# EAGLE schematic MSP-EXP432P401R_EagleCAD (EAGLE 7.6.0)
AUTHOR: Mike Stein; REV: 2.1

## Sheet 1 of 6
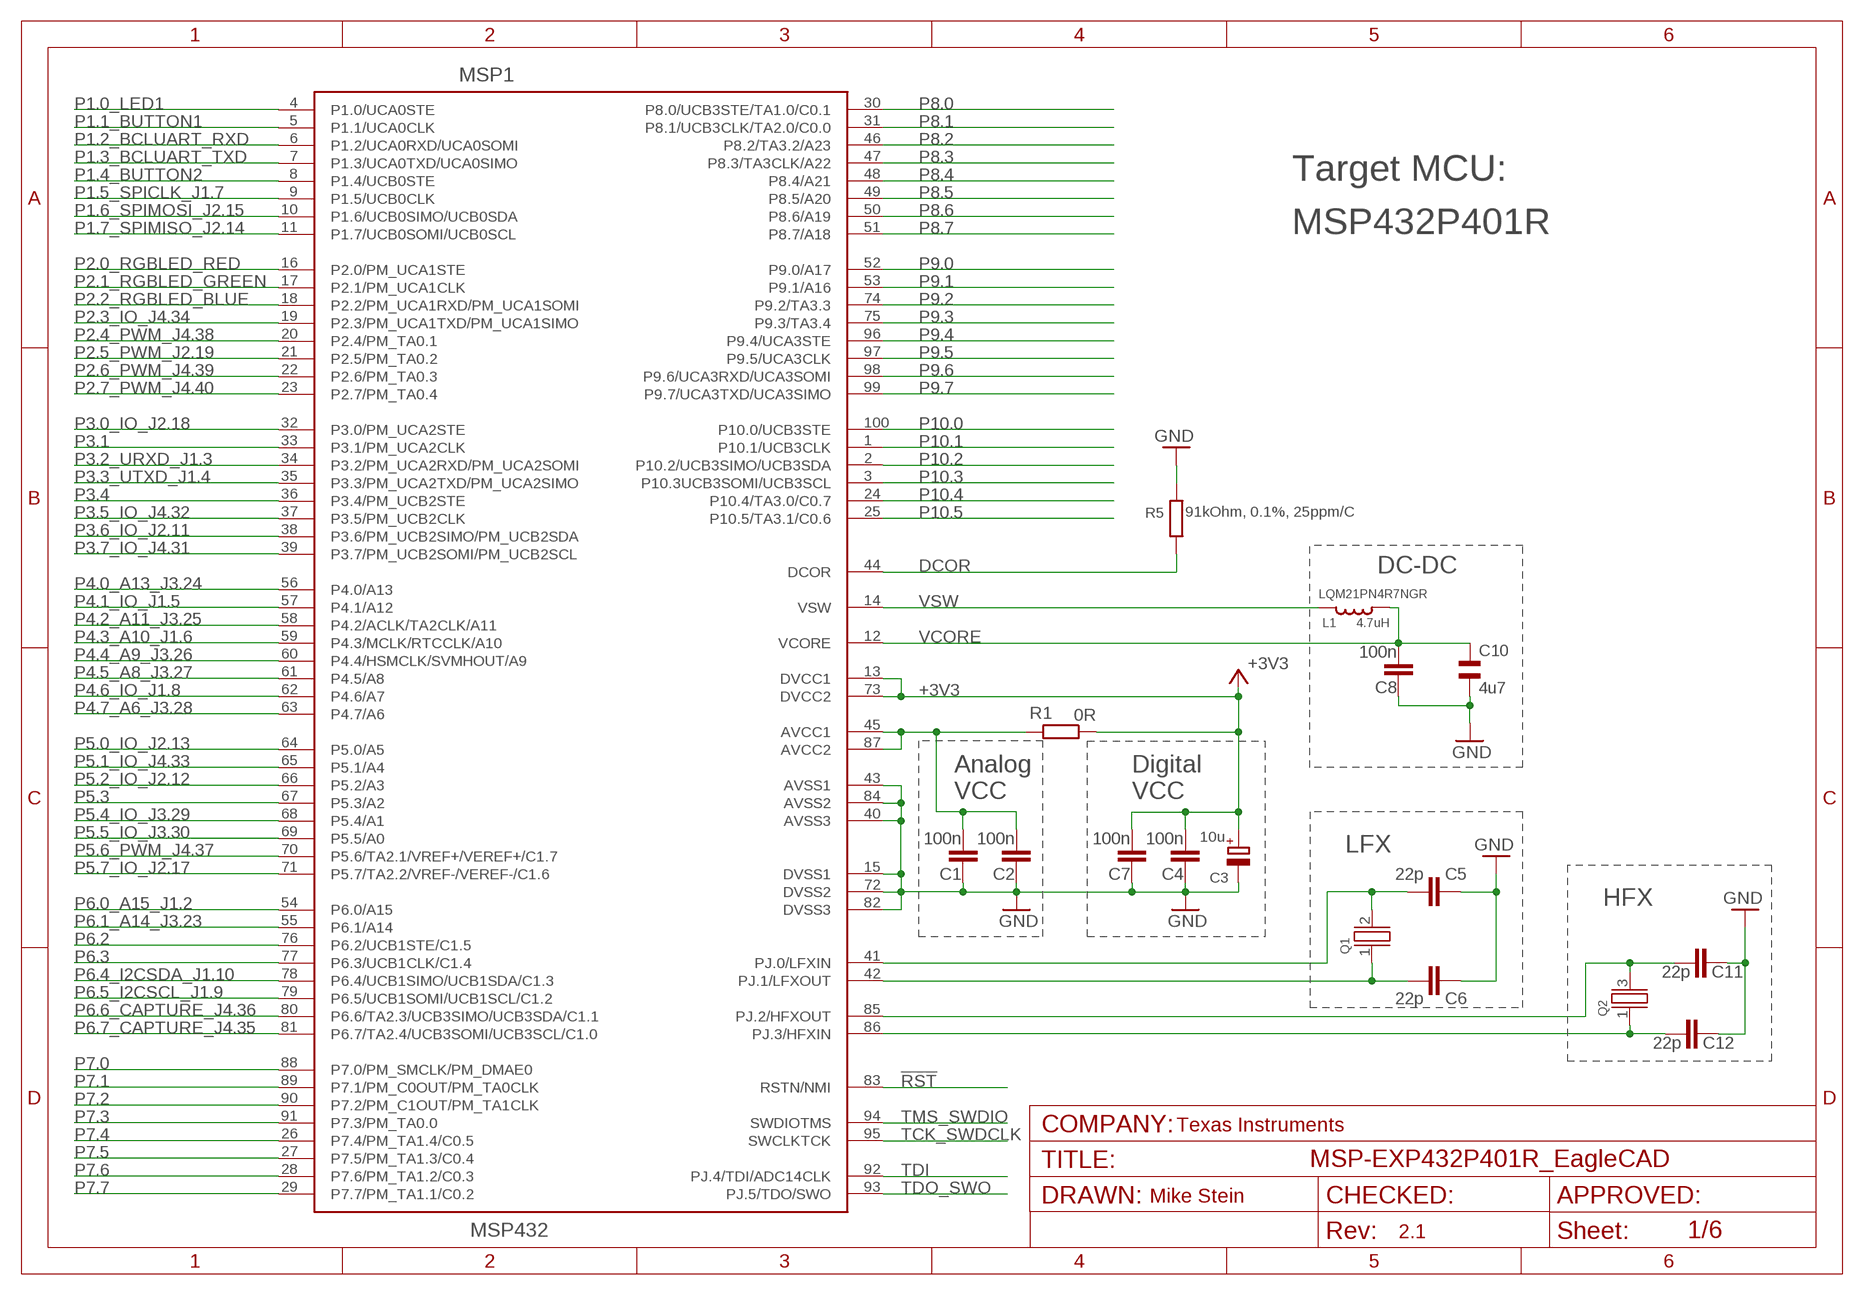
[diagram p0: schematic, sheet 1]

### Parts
C1  100n  C-EUCM0402  [0402]
C2  100n  C-EUCM0402  [0402]
C3  10u  CPOL-EUA/3216-18R  [A/3216-18R]
C4  100n  C-EUCM0402  [0402]
C5  22p  C-EUCM0402  [0402]
C6  22p  C-EUCM0402  [0402]
C7  100n  C-EUCM0402  [0402]
C8  100n  C-EUCM0402  [0402]
C10  4u7  CSMD0805  [CSMD0805]
C11  22p  C-EUCM0402  [0402]
C12  22p  C-EUCM0402  [0402]
L1  4.7uH  LQM2MP_G0  [0806]
MSP1  MSP432  [PZ100]
Q1  CRYSTALLF_GENERAL  [LF_XTAL]
Q2  CRYSTALEPSON_FA-238  [FA-238]
R1  0R  R-EU_RM0402  [0402]
R5  91kOhm, 0.1%, 25ppm/C  R_0805  [0805]

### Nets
!RST: MSP1.83(RSTN/NMI) ; also sheet 2,3
+3V3: C3.+ C4.1 C7.1 MSP1.13(DVCC1) MSP1.73(DVCC2) R1.1 ; also sheet 2,3
DCOR: MSP1.44(DCOR) R5.1
N$6: C1.1 C2.1 MSP1.45(AVCC1) MSP1.87(AVCC2) R1.2
N$34: C6.1 MSP1.42(PJ.1/LFXOUT) Q1.1
N$38: C5.1 MSP1.41(PJ.0/LFXIN) Q1.2
P1.0_LED1: MSP1.4(P1.0/UCA0STE) ; also sheet 2
P1.1_BUTTON1: MSP1.5(P1.1/UCA0CLK) ; also sheet 2
P1.2_BCLUART_RXD: MSP1.6(P1.2/UCA0RXD/UCA0SOMI) ; also sheet 3
P1.3_BCLUART_TXD: MSP1.7(P1.3/UCA0TXD/UCA0SIMO) ; also sheet 3
P1.4_BUTTON2: MSP1.8(P1.4/UCB0STE) ; also sheet 2
P1.5_SPICLK_J1.7: MSP1.9(P1.5/UCB0CLK) ; also sheet 3
P1.6_SPIMOSI_J2.15: MSP1.10(P1.6/UCB0SIMO/UCB0SDA) ; also sheet 3
P1.7_SPIMISO_J2.14: MSP1.11(P1.7/UCB0SOMI/UCB0SCL) ; also sheet 3
P2.0_RGBLED_RED: MSP1.16(P2.0/PM_UCA1STE) ; also sheet 2
P2.1_RGBLED_GREEN: MSP1.17(P2.1/PM_UCA1CLK) ; also sheet 2
P2.2_RGBLED_BLUE: MSP1.18(P2.2/PM_UCA1RXD/PM_UCA1SOMI) ; also sheet 2
P2.3_IO_J4.34: MSP1.19(P2.3/PM_UCA1TXD/PM_UCA1SIMO) ; also sheet 3
P2.4_PWM_J4.38: MSP1.20(P2.4/PM_TA0.1) ; also sheet 3
P2.5_PWM_J2.19: MSP1.21(P2.5/PM_TA0.2) ; also sheet 3
P2.6_PWM_J4.39: MSP1.22(P2.6/PM_TA0.3) ; also sheet 3
P2.7_PWM_J4.40: MSP1.23(P2.7/PM_TA0.4) ; also sheet 3
P3.0_IO_J2.18: MSP1.32(P3.0/PM_UCA2STE) ; also sheet 3
P3.1: MSP1.33(P3.1/PM_UCA2CLK)
P3.2_URXD_J1.3: MSP1.34(P3.2/PM_UCA2RXD/PM_UCA2SOMI) ; also sheet 3
P3.3_UTXD_J1.4: MSP1.35(P3.3/PM_UCA2TXD/PM_UCA2SIMO) ; also sheet 3
P3.4: MSP1.36(P3.4/PM_UCB2STE)
P3.5_IO_J4.32: MSP1.37(P3.5/PM_UCB2CLK) ; also sheet 3
P3.6_IO_J2.11: MSP1.38(P3.6/PM_UCB2SIMO/PM_UCB2SDA) ; also sheet 3
P3.7_IO_J4.31: MSP1.39(P3.7/PM_UCB2SOMI/PM_UCB2SCL) ; also sheet 3
P4.0_A13_J3.24: MSP1.56(P4.0/A13) ; also sheet 3
P4.1_IO_J1.5: MSP1.57(P4.1/A12) ; also sheet 3
P4.2_A11_J3.25: MSP1.58(P4.2/ACLK/TA2CLK/A11) ; also sheet 3
P4.3_A10_J1.6: MSP1.59(P4.3/MCLK/RTCCLK/A10) ; also sheet 3
P4.4_A9_J3.26: MSP1.60(P4.4/HSMCLK/SVMHOUT/A9) ; also sheet 3
P4.5_A8_J3.27: MSP1.61(P4.5/A8) ; also sheet 3
P4.6_IO_J1.8: MSP1.62(P4.6/A7) ; also sheet 3
P4.7_A6_J3.28: MSP1.63(P4.7/A6) ; also sheet 3
P5.0_IO_J2.13: MSP1.64(P5.0/A5) ; also sheet 3
P5.1_IO_J4.33: MSP1.65(P5.1/A4) ; also sheet 3
P5.2/XT2IN: C12.1 MSP1.86(PJ.3/HFXIN) Q2.1
P5.2_IO_J2.12: MSP1.66(P5.2/A3) ; also sheet 3
P5.3: MSP1.67(P5.3/A2) ; also sheet 3
P5.3/XT2OUT: C11.1 MSP1.85(PJ.2/HFXOUT) Q2.3
P5.4_IO_J3.29: MSP1.68(P5.4/A1) ; also sheet 3
P5.5_IO_J3.30: MSP1.69(P5.5/A0) ; also sheet 3
P5.6_PWM_J4.37: MSP1.70(P5.6/TA2.1/VREF+/VEREF+/C1.7) ; also sheet 3
P5.7_IO_J2.17: MSP1.71(P5.7/TA2.2/VREF-/VEREF-/C1.6) ; also sheet 3
P6.0_A15_J1.2: MSP1.54(P6.0/A15) ; also sheet 3
P6.1_A14_J3.23: MSP1.55(P6.1/A14) ; also sheet 3
P6.2: MSP1.76(P6.2/UCB1STE/C1.5) ; also sheet 3
P6.3: MSP1.77(P6.3/UCB1CLK/C1.4) ; also sheet 3
P6.4_I2CSDA_J1.10: MSP1.78(P6.4/UCB1SIMO/UCB1SDA/C1.3) ; also sheet 3
P6.5_I2CSCL_J1.9: MSP1.79(P6.5/UCB1SOMI/UCB1SCL/C1.2) ; also sheet 3
P6.6_CAPTURE_J4.36: MSP1.80(P6.6/TA2.3/UCB3SIMO/UCB3SDA/C1.1) ; also sheet 3
P6.7_CAPTURE_J4.35: MSP1.81(P6.7/TA2.4/UCB3SOMI/UCB3SCL/C1.0) ; also sheet 3
P7.0: MSP1.88(P7.0/PM_SMCLK/PM_DMAE0) ; also sheet 3
P7.1: MSP1.89(P7.1/PM_C0OUT/PM_TA0CLK) ; also sheet 3
P7.2: MSP1.90(P7.2/PM_C1OUT/PM_TA1CLK) ; also sheet 3
P7.3: MSP1.91(P7.3/PM_TA0.0) ; also sheet 3
P7.4: MSP1.26(P7.4/PM_TA1.4/C0.5) ; also sheet 3
P7.5: MSP1.27(P7.5/PM_TA1.3/C0.4) ; also sheet 3
P7.6: MSP1.28(P7.6/PM_TA1.2/C0.3) ; also sheet 3
P7.7: MSP1.29(P7.7/PM_TA1.1/C0.2) ; also sheet 3
P8.0: MSP1.30(P8.0/UCB3STE/TA1.0/C0.1) ; also sheet 3
P8.1: MSP1.31(P8.1/UCB3CLK/TA2.0/C0.0)
P8.2: MSP1.46(P8.2/TA3.2/A23) ; also sheet 3
P8.3: MSP1.47(P8.3/TA3CLK/A22) ; also sheet 3
P8.4: MSP1.48(P8.4/A21) ; also sheet 3
P8.5: MSP1.49(P8.5/A20) ; also sheet 3
P8.6: MSP1.50(P8.6/A19) ; also sheet 3
P8.7: MSP1.51(P8.7/A18) ; also sheet 3
P9.0: MSP1.52(P9.0/A17) ; also sheet 3
P9.1: MSP1.53(P9.1/A16) ; also sheet 3
P9.2: MSP1.74(P9.2/TA3.3) ; also sheet 3
P9.3: MSP1.75(P9.3/TA3.4) ; also sheet 3
P9.4: MSP1.96(P9.4/UCA3STE) ; also sheet 3
P9.5: MSP1.97(P9.5/UCA3CLK) ; also sheet 3
P9.6: MSP1.98(P9.6/UCA3RXD/UCA3SOMI) ; also sheet 3
P9.7: MSP1.99(P9.7/UCA3TXD/UCA3SIMO) ; also sheet 3
P10.0: MSP1.100(P10.0/UCB3STE) ; also sheet 3
P10.1: MSP1.1(P10.1/UCB3CLK) ; also sheet 3
P10.2: MSP1.2(P10.2/UCB3SIMO/UCB3SDA) ; also sheet 3
P10.3: MSP1.3(P10.3UCB3SOMI/UCB3SCL) ; also sheet 3
P10.4: MSP1.24(P10.4/TA3.0/C0.7) ; also sheet 3
P10.5: MSP1.25(P10.5/TA3.1/C0.6) ; also sheet 3
TCK_SWDCLK: MSP1.95(SWCLKTCK) ; also sheet 3
TDI: MSP1.92(PJ.4/TDI/ADC14CLK) ; also sheet 3
TDO_SWO: MSP1.93(PJ.5/TDO/SWO) ; also sheet 3
TMS_SWDIO: MSP1.94(SWDIOTMS) ; also sheet 3
VCORE: C8.1 C10.1 L1.1 MSP1.12(VCORE)
VSW: L1.2 MSP1.14(VSW)
XDS-GND: C1.2 C2.2 C3.- C4.2 C5.2 C6.2 C7.2 C8.2 C10.2 C11.2 C12.2 MSP1.15(DVSS1) MSP1.40(AVSS3) MSP1.43(AVSS1) MSP1.72(DVSS2) MSP1.82(DVSS3) MSP1.84(AVSS2) R5.2 ; supply symbol labelled GND ; also sheet 2,3

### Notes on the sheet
- Target MCU:
- MSP432P401R
- DC-DC
- LQM21PN4R7NGR
- Analog | Digital
- VCC | VCC
- LFX
- HFX
- Texas Instruments

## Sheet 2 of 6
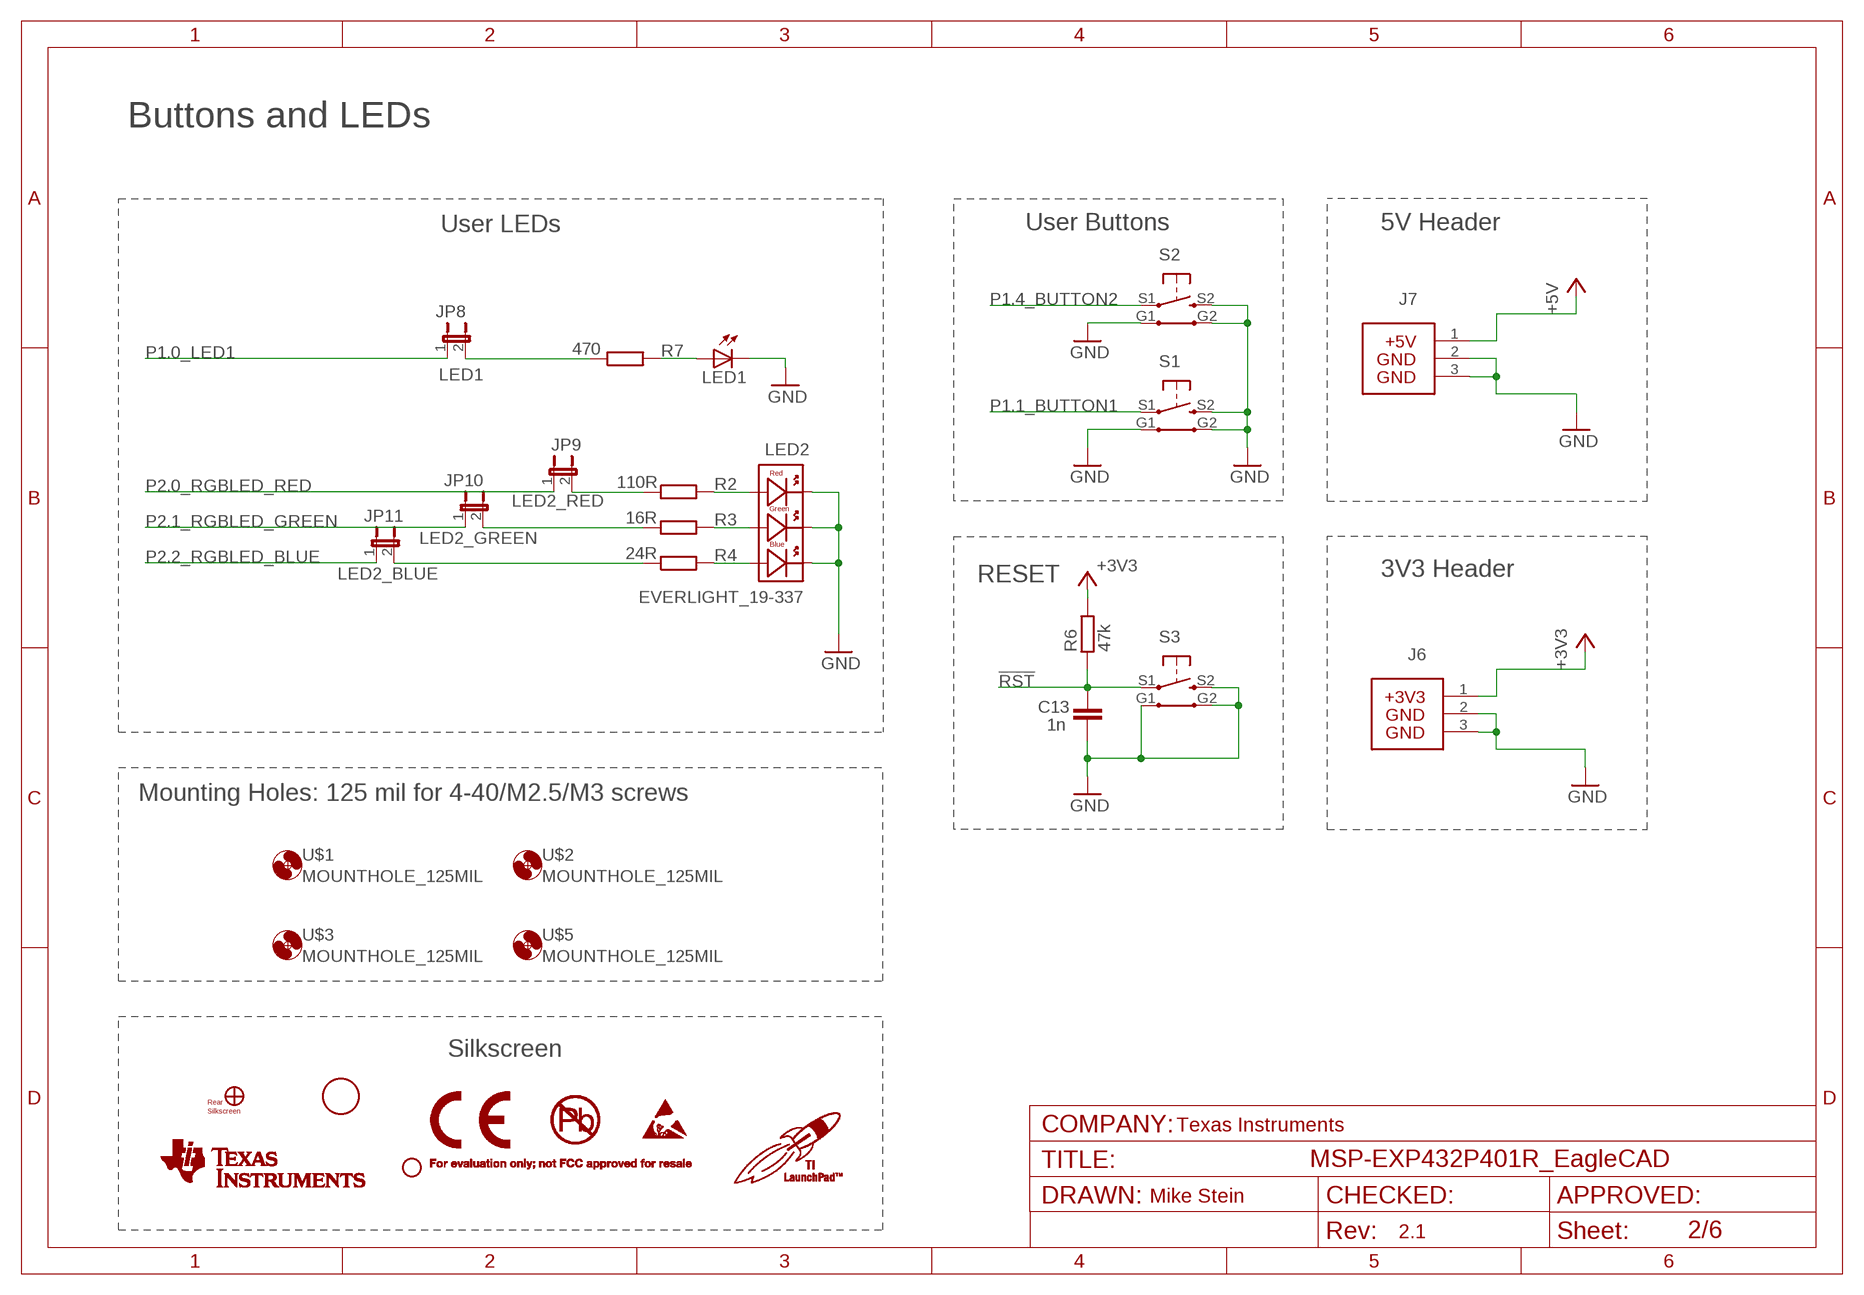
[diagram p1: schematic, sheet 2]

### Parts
C13  1n  C-EUCM0402  [0402]
J6  HEADER 1X03  BP_HEADERS_PWR_3V3100-TH  [3PIN_PWR_3V3]
J7  BP_HEADERS_PWR_5V  [3PIN_PWR_5V]
JP8  LED1  JP1M  [JP1M]
JP9  LED2_RED  JP1M  [JP1M]
JP10  LED2_GREEN  JP1M  [JP1M]
JP11  LED2_BLUE  JP1M  [JP1M]
LED1  LEDCHIPLED_0603  [CHIPLED_0603]
LED2  EVERLIGHT_19-337  [RGB_LED]
R2  110R  R-EU_RM0402  [0402]
R3  16R  R-EU_RM0402  [0402]
R4  24R  R-EU_RM0402  [0402]
R6  47k  R-EU_RM0402  [0402]
R7  470  R-EU_RM0402  [0402]
S1  TS-1188E  [TS-1188E]
S2  TS-1188E  [TS-1188E]
S3  TS-1188E  [TS-1188E]
U$1  MOUNTHOLE_125MIL  [MOUNTHOLE_125MIL]
U$2  MOUNTHOLE_125MIL  [MOUNTHOLE_125MIL]
U$3  MOUNTHOLE_125MIL  [MOUNTHOLE_125MIL]
U$5  MOUNTHOLE_125MIL  [MOUNTHOLE_125MIL]
U$7  MIKE_TM  [MIKE_TM]
U$8  P401R_REARSILK_REV2_1  [P401R_REARSILK_REV2_1]
U$9  REAR_TILOGO  [REAR_TILOGO]
U$10  COMPLIANCE_SUITESYMBOLONLY  [EVM_COMPLIANCESUITE_SYMBOLONLY]
U$11  COMPLIANCE_FCC_TEXTREAR  [COMPLIANCE_FCC_TEXT]
U$12  LOGO-ROCKET  [LOGO-ROCKET]
U$13  P401R_SILKLABEL  [SILKLABELUPDATED]

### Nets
!RST: C13.1 R6.1 S3.S1(P) ; also sheet 1,3
+3V3: J6.1 R6.2 ; also sheet 1,3
+5V [Power]: J7.1 ; also sheet 3
N$8: JP9.2 R2.1
N$9: LED2.5(RA) R2.2
N$10: LED2.6(GA) R3.2
N$11: LED2.4(BA) R4.2
N$17: LED1.A R7.2
N$19: JP10.2 R3.1
N$25: JP11.2 R4.1
N$29: JP8.2 R7.1
P1.0_LED1: JP8.1 ; also sheet 1
P1.1_BUTTON1: S1.S1(P) ; also sheet 1
P1.4_BUTTON2: S2.S1(P) ; also sheet 1
P2.0_RGBLED_RED: JP9.1 ; also sheet 1
P2.1_RGBLED_GREEN: JP10.1 ; also sheet 1
P2.2_RGBLED_BLUE: JP11.1 ; also sheet 1
XDS-GND: C13.2 J6.2 J6.3 J7.2 J7.3 LED1.C LED2.1(BC) LED2.2(RC) LED2.3(GC) S1.G1 S1.G2 S1.S2(S) S2.G1 S2.G2 S2.S2(S) S3.G1 S3.G2 S3.S2(S) ; supply symbol labelled GND ; also sheet 1,3

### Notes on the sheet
- Buttons and LEDs
- User LEDs | User Buttons | 5V Header
- RESET | 3V3 Header
- Mounting Holes: 125 mil for 4-40/M2.5/M3 screws
- Silkscreen
- Texas Instruments

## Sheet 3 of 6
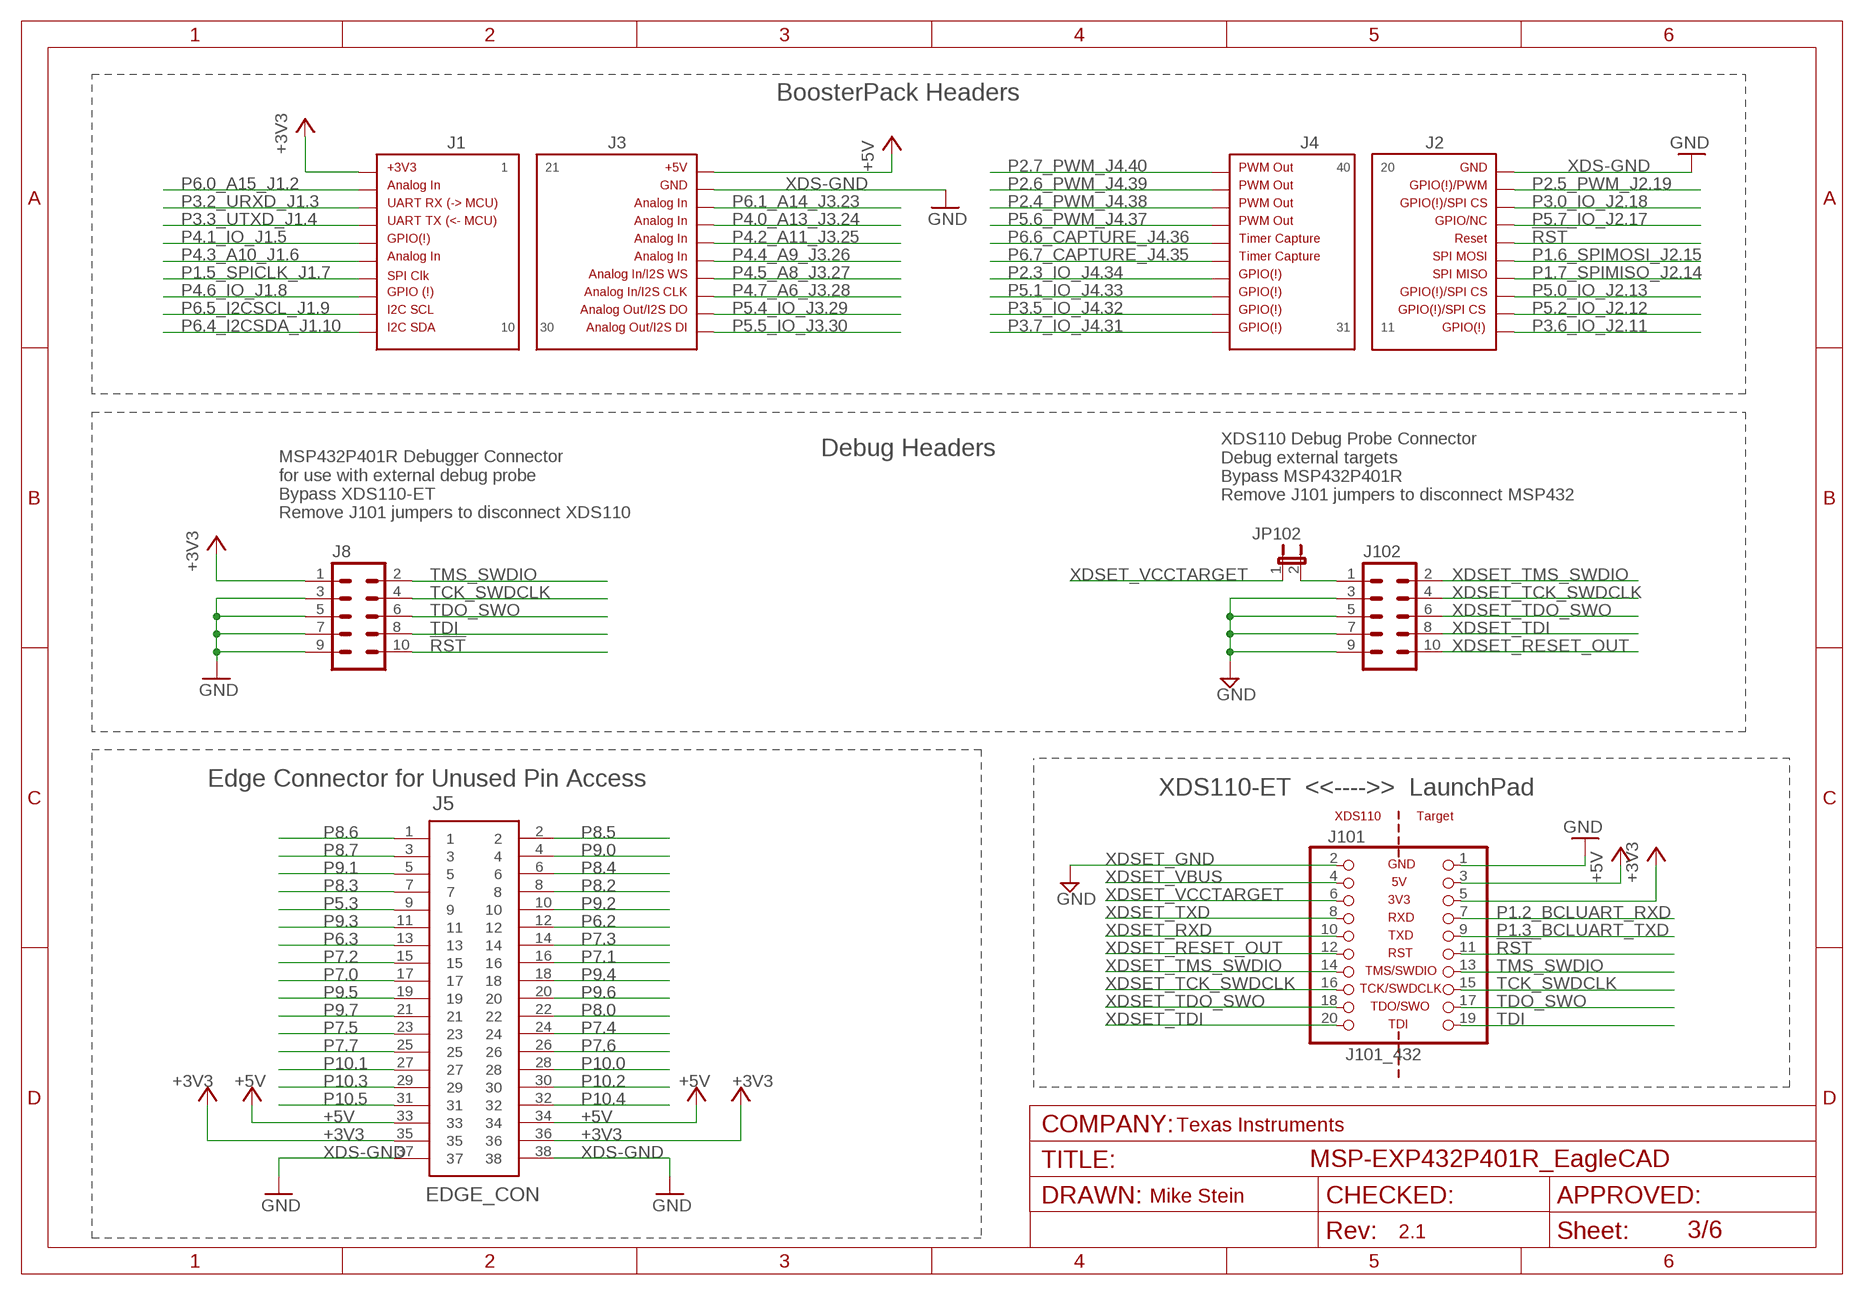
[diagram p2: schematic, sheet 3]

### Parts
J1  HEADER1X10-J1SILK_LABELS  [J1]
J2  HEADER1X10-J2SILK_LABELS  [J2]
J3  HEADER1X10-J3  [J3]
J4  HEADER1X10-J4SILK_LABELS  [J4]
J5  EDGE_CON  [BOTTOM_CONNECTOR]
J8  DEBUG_ARM-10  [ARM-10]
J101  J101_432  [J101_432]
J102  DEBUG_ARM-10  [ARM-10]
JP102  JP1M  [JP1M]

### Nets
!RST: J2.16 J8.10 J101.11 ; also sheet 1,2
+3V3: J1.1 J5.35 J5.36 J8.1 J101.5 ; also sheet 1,2
+5V [Power]: J3.21 J5.33 J5.34 J101.3 ; also sheet 2
N$1: J102.1 JP102.2
P1.2_BCLUART_RXD: J101.7 ; also sheet 1
P1.3_BCLUART_TXD: J101.9 ; also sheet 1
P1.5_SPICLK_J1.7: J1.7 ; also sheet 1
P1.6_SPIMOSI_J2.15: J2.15 ; also sheet 1
P1.7_SPIMISO_J2.14: J2.14 ; also sheet 1
P2.3_IO_J4.34: J4.34 ; also sheet 1
P2.4_PWM_J4.38: J4.38 ; also sheet 1
P2.5_PWM_J2.19: J2.19 ; also sheet 1
P2.6_PWM_J4.39: J4.39 ; also sheet 1
P2.7_PWM_J4.40: J4.40 ; also sheet 1
P3.0_IO_J2.18: J2.18 ; also sheet 1
P3.2_URXD_J1.3: J1.3 ; also sheet 1
P3.3_UTXD_J1.4: J1.4 ; also sheet 1
P3.5_IO_J4.32: J4.32 ; also sheet 1
P3.6_IO_J2.11: J2.11 ; also sheet 1
P3.7_IO_J4.31: J4.31 ; also sheet 1
P4.0_A13_J3.24: J3.24 ; also sheet 1
P4.1_IO_J1.5: J1.5 ; also sheet 1
P4.2_A11_J3.25: J3.25 ; also sheet 1
P4.3_A10_J1.6: J1.6 ; also sheet 1
P4.4_A9_J3.26: J3.26 ; also sheet 1
P4.5_A8_J3.27: J3.27 ; also sheet 1
P4.6_IO_J1.8: J1.8 ; also sheet 1
P4.7_A6_J3.28: J3.28 ; also sheet 1
P5.0_IO_J2.13: J2.13 ; also sheet 1
P5.1_IO_J4.33: J4.33 ; also sheet 1
P5.2_IO_J2.12: J2.12 ; also sheet 1
P5.3: J5.9 ; also sheet 1
P5.4_IO_J3.29: J3.29 ; also sheet 1
P5.5_IO_J3.30: J3.30 ; also sheet 1
P5.6_PWM_J4.37: J4.37 ; also sheet 1
P5.7_IO_J2.17: J2.17 ; also sheet 1
P6.0_A15_J1.2: J1.2 ; also sheet 1
P6.1_A14_J3.23: J3.23 ; also sheet 1
P6.2: J5.12 ; also sheet 1
P6.3: J5.13 ; also sheet 1
P6.4_I2CSDA_J1.10: J1.10 ; also sheet 1
P6.5_I2CSCL_J1.9: J1.9 ; also sheet 1
P6.6_CAPTURE_J4.36: J4.36 ; also sheet 1
P6.7_CAPTURE_J4.35: J4.35 ; also sheet 1
P7.0: J5.17 ; also sheet 1
P7.1: J5.16 ; also sheet 1
P7.2: J5.15 ; also sheet 1
P7.3: J5.14 ; also sheet 1
P7.4: J5.24 ; also sheet 1
P7.5: J5.23 ; also sheet 1
P7.6: J5.26 ; also sheet 1
P7.7: J5.25 ; also sheet 1
P8.0: J5.22 ; also sheet 1
P8.2: J5.8 ; also sheet 1
P8.3: J5.7 ; also sheet 1
P8.4: J5.6 ; also sheet 1
P8.5: J5.2 ; also sheet 1
P8.6: J5.1 ; also sheet 1
P8.7: J5.3 ; also sheet 1
P9.0: J5.4 ; also sheet 1
P9.1: J5.5 ; also sheet 1
P9.2: J5.10 ; also sheet 1
P9.3: J5.11 ; also sheet 1
P9.4: J5.18 ; also sheet 1
P9.5: J5.19 ; also sheet 1
P9.6: J5.20 ; also sheet 1
P9.7: J5.21 ; also sheet 1
P10.0: J5.28 ; also sheet 1
P10.1: J5.27 ; also sheet 1
P10.2: J5.30 ; also sheet 1
P10.3: J5.29 ; also sheet 1
P10.4: J5.32 ; also sheet 1
P10.5: J5.31 ; also sheet 1
TCK_SWDCLK: J8.4 J101.15 ; also sheet 1
TDI: J8.8 J101.19 ; also sheet 1
TDO_SWO: J8.6 J101.17 ; also sheet 1
TMS_SWDIO: J8.2 J101.13 ; also sheet 1
XDS-GND: J2.20 J3.22 J5.37 J5.38 J8.3 J8.5 J8.7 J8.9 J101.1 ; supply symbol labelled GND ; also sheet 1,2
XDSET_GND: J101.2 J102.3 J102.5 J102.7 J102.9 ; supply symbol labelled GND ; also sheet 4,5,6
XDSET_RESET_OUT: J101.12 J102.10 ; also sheet 4
XDSET_RXD: J101.10 ; also sheet 4
XDSET_TCK_SWDCLK: J101.16 J102.4 ; also sheet 4
XDSET_TDI: J101.20 J102.8 ; also sheet 4
XDSET_TDO_SWO: J101.18 J102.6 ; also sheet 4
XDSET_TMS_SWDIO: J101.14 J102.2 ; also sheet 4
XDSET_TXD: J101.8 ; also sheet 4
XDSET_VBUS: J101.4 ; also sheet 4,5,6
XDSET_VCCTARGET: J101.6 JP102.1 ; also sheet 5

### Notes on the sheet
- BoosterPack Headers
- Debug Headers
- XDS110 Debug Probe Connector
  Debug external targets
  Bypass MSP432P401R
  Remove J101 jumpers to disconnect MSP432
- MSP432P401R Debugger Connector
  for use with external debug probe
  Bypass XDS110-ET
  Remove J101 jumpers to disconnect XDS110
- Edge Connector for Unused Pin Access
- XDS110-ET  <<---->>  LaunchPad
- Texas Instruments

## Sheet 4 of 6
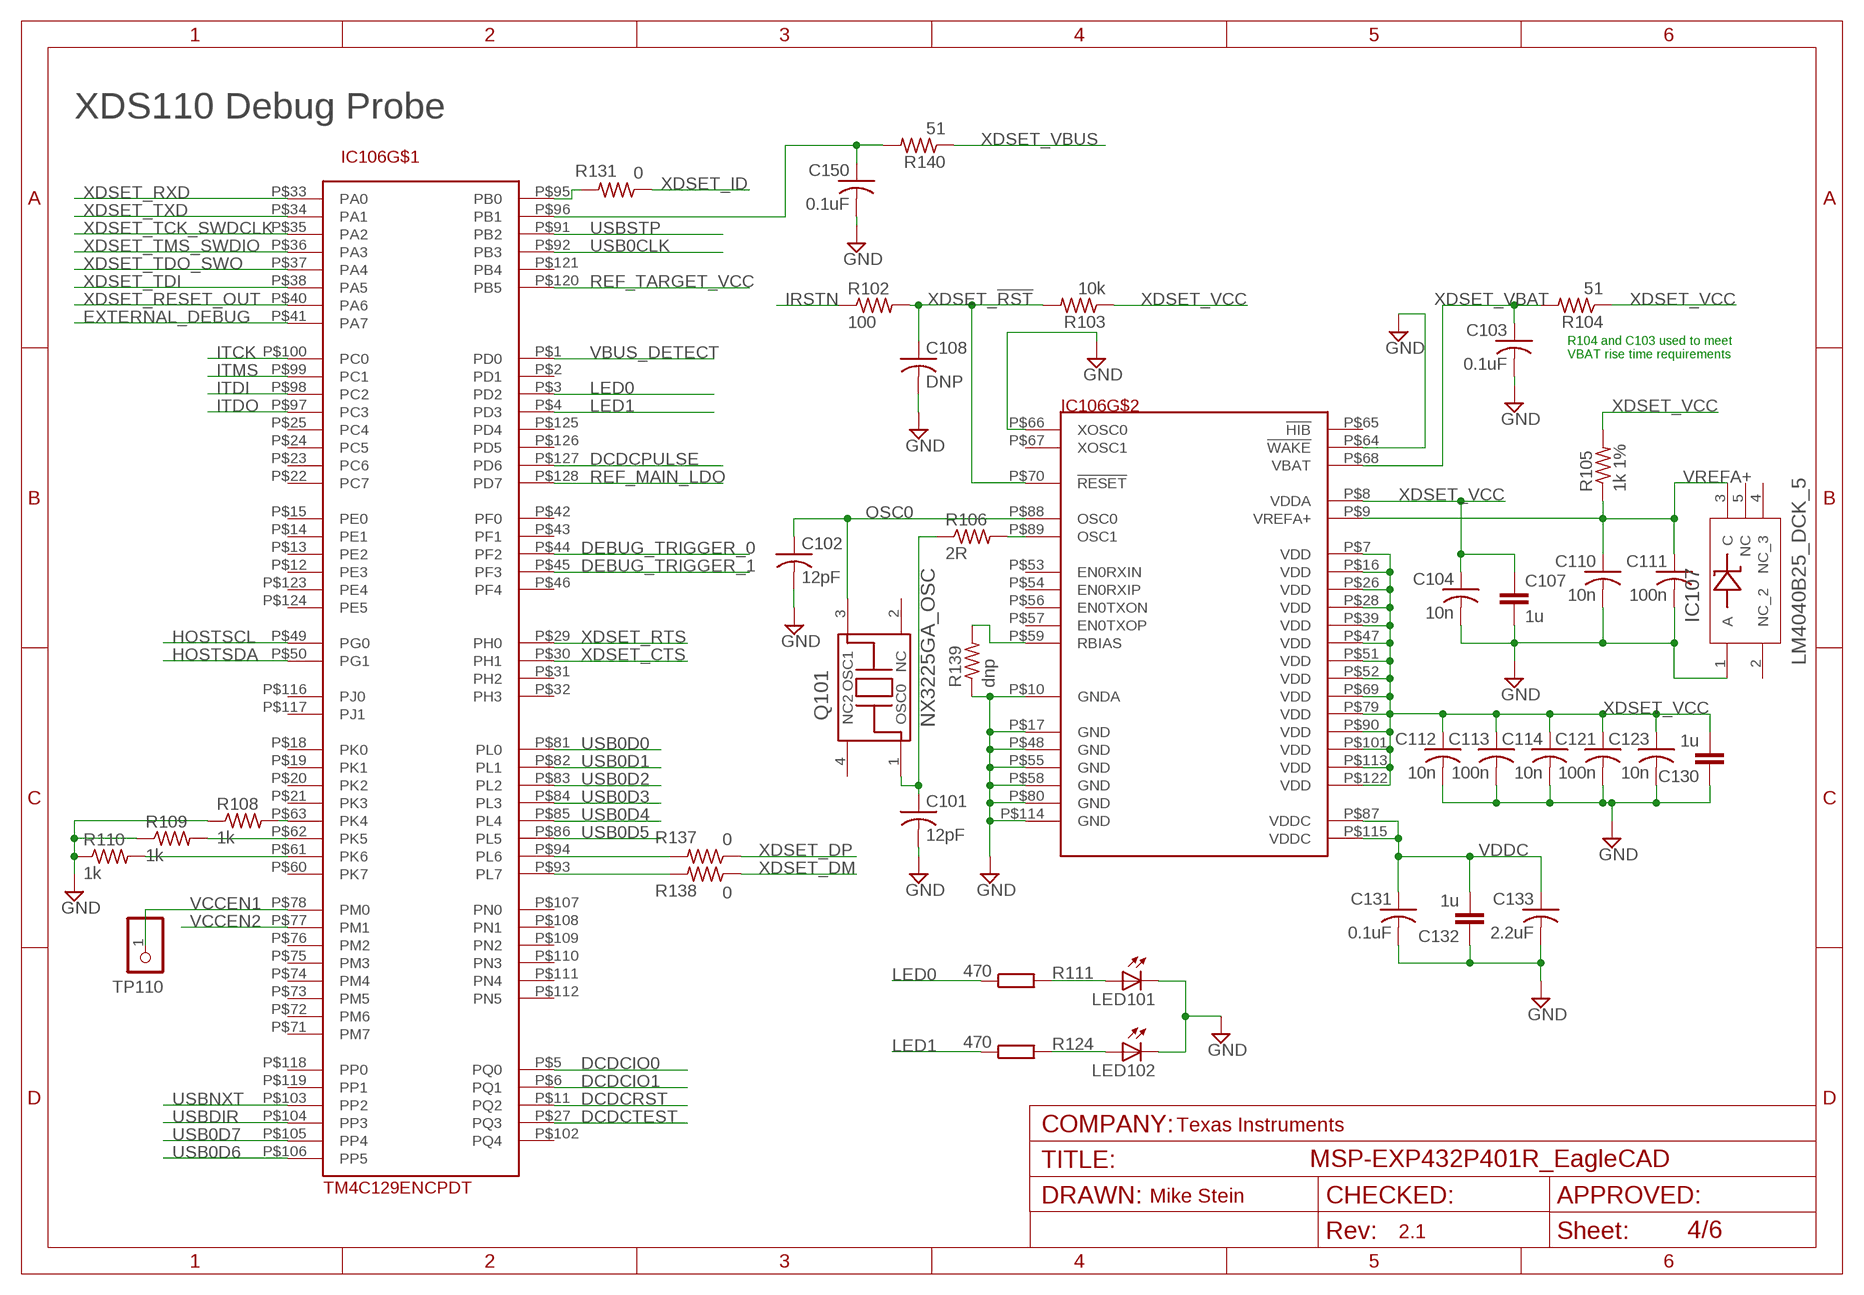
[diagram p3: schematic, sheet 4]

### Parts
C101  12pF  C-USC0402  [C0402]
C102  12pF  C-USC0402  [C0402]
C103  0.1uF  C-USC0402  [C0402]
C104  10n  C-USC0402  [C0402]
C107  1u  C-EUC0603  [C0603]
C108  DNP  C-USC0402  [C0402]
C110  10n  C-USC0402  [C0402]
C111  100n  C-USC0402  [C0402]
C112  10n  C-USC0402  [C0402]
C113  100n  C-USC0402  [C0402]
C114  10n  C-USC0402  [C0402]
C121  100n  C-USC0402  [C0402]
C123  10n  C-USC0402  [C0402]
C130  1u  C-EUC0603  [C0603]
C131  0.1uF  C-USC0402  [C0402]
C132  1u  C-EUC0603  [C0603]
C133  2.2uF  C-USC0603K  [C0603K]
C150  0.1uF  C-USC0402  [C0402]
IC106  TM4C129ENCPDT  [TQFP-128]
IC107  LM4040B25_DCK_5  [DCK5]
LED101  LEDCHIPLED_0603  [CHIPLED_0603]
LED102  LEDCHIPLED_0603  [CHIPLED_0603]
Q101  NX3225GA_OSC  [NX3225GA]
R102  100  R-US_R0402  [R0402]
R103  10k  R-US_R0402  [R0402]
R104  51  R-US_R0402  [R0402]
R105  1k 1%  R-US_R0402  [R0402]
R106  2R  R-US_R0402  [R0402]
R108  1k  R-US_R0402  [R0402]
R109  1k  R-US_R0402  [R0402]
R110  1k  R-US_R0402  [R0402]
R111  470  R-EU_RM0402  [0402]
R124  470  R-EU_RM0402  [0402]
R131  0  R-US_R0402  [R0402]
R137  0  R-US_R0402  [R0402]
R138  0  R-US_R0402  [R0402]
R139  dnp  R-US_R0402  [R0402]
R140  51  R-US_R0402  [R0402]
TP110  TEST_PIN2  PINHD-1X1  [1X01]

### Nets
DCDCIO0: IC106.P$5(PQ0) ; also sheet 5
DCDCIO1: IC106.P$6(PQ1) ; also sheet 5
DCDCPULSE: IC106.P$127(PD6) ; also sheet 5
DCDCRST: IC106.P$11(PQ2) ; also sheet 5,6
DCDCTEST: IC106.P$27(PQ3) ; also sheet 5,6
DEBUG_TRIGGER_0: IC106.P$44(PF2)
DEBUG_TRIGGER_1: IC106.P$45(PF3)
EXTERNAL_DEBUG: IC106.P$41(PA7)
HOSTSCL: IC106.P$49(PG0) ; also sheet 5
HOSTSDA: IC106.P$50(PG1) ; also sheet 5
IRSTN: R102.1 ; also sheet 6
ITCK: IC106.P$100(PC0) ; also sheet 6
ITDI: IC106.P$98(PC2) ; also sheet 6
ITDO: IC106.P$97(PC3) ; also sheet 6
ITMS: IC106.P$99(PC1) ; also sheet 6
LED0: IC106.P$3(PD2) R111.1
LED1: IC106.P$4(PD3) R124.1
N$3: IC106.P$63(PK4) R108.2
N$4: LED102.A R124.2
N$7: LED101.A R111.2
N$21: IC106.P$93(PL7) R138.2
N$22: IC106.P$61(PK6) R110.2
N$23: IC106.P$95(PB0) R131.2
N$27: IC106.P$62(PK5) R109.2
N$47: IC106.P$59(RBIAS) R139.2
OSC0: C102.1 IC106.P$88(OSC0) Q101.3(OSC1)
OSC1: IC106.P$89(OSC1) R106.2
OSC1_R: C101.1 Q101.1(OSC0) R106.1
P96VBUS: C150.1 IC106.P$96(PB1) R140.2
REF_MAIN_LDO: IC106.P$128(PD7) ; also sheet 5
REF_TARGET_VCC: IC106.P$120(PB5) ; also sheet 5
USB0CLK: IC106.P$92(PB3)
USB0D0: IC106.P$81(PL0)
USB0D1: IC106.P$82(PL1)
USB0D2: IC106.P$83(PL2)
USB0D3: IC106.P$84(PL3)
USB0D4: IC106.P$85(PL4)
USB0D5: IC106.P$86(PL5)
USB0D6: IC106.P$106(PP5)
USB0D7: IC106.P$105(PP4)
USBDIR: IC106.P$104(PP3)
USBNXT: IC106.P$103(PP2)
USBSTP: IC106.P$91(PB2)
VBUS_DETECT: IC106.P$1(PD0) ; also sheet 6
VCCEN1: IC106.P$78(PM0) TP110.1 ; also sheet 5
VCCEN2: IC106.P$77(PM1)
VDDC: C131.1 C132.2 C133.1 IC106.P$87(VDDC) IC106.P$115(VDDC)
VREFA+: C110.1 C111.1 IC106.P$9(VREFA+) IC107.3(C) R105.1
XDSET_!RST: C108.1 IC106.P$70(!RESET) R102.2 R103.2
XDSET_CTS: IC106.P$30(PH1)
XDSET_DM: R138.1 ; also sheet 6
XDSET_DP: R137.1 ; also sheet 6
XDSET_DPR: IC106.P$94(PL6) R137.2
XDSET_GND: C101.2 C102.2 C103.2 C104.2 C107.2 C108.2 C110.2 C111.2 C112.2 C113.2 C114.2 C121.2 C123.2 C130.1 C131.2 C132.1 C133.2 C150.2 IC106.P$10(GNDA) IC106.P$17(GND) IC106.P$48(GND) IC106.P$55(GND) IC106.P$58(GND) IC106.P$64(!WAKE) IC106.P$66(XOSC0) IC106.P$80(GND) IC106.P$114(GND) IC107.1(A) LED101.C LED102.C R108.1 R109.1 R110.1 R139.1 ; supply symbol labelled GND ; also sheet 3,5,6
XDSET_ID: R131.1 ; also sheet 6
XDSET_RESET_OUT: IC106.P$40(PA6) ; also sheet 3
XDSET_RTS: IC106.P$29(PH0)
XDSET_RXD: IC106.P$33(PA0) ; also sheet 3
XDSET_TCK_SWDCLK: IC106.P$35(PA2) ; also sheet 3
XDSET_TDI: IC106.P$38(PA5) ; also sheet 3
XDSET_TDO_SWO: IC106.P$37(PA4) ; also sheet 3
XDSET_TMS_SWDIO: IC106.P$36(PA3) ; also sheet 3
XDSET_TXD: IC106.P$34(PA1) ; also sheet 3
XDSET_VBAT: C103.1 IC106.P$68(VBAT) R104.2
XDSET_VBUS: R140.1 ; also sheet 3,5,6
XDSET_VCC: C104.1 C107.1 C112.1 C113.1 C114.1 C121.1 C123.1 C130.2 IC106.P$7(VDD) IC106.P$8(VDDA) IC106.P$16(VDD) IC106.P$26(VDD) IC106.P$28(VDD) IC106.P$39(VDD) IC106.P$47(VDD) IC106.P$51(VDD) IC106.P$52(VDD) IC106.P$69(VDD) IC106.P$79(VDD) IC106.P$90(VDD) IC106.P$101(VDD) IC106.P$113(VDD) IC106.P$122(VDD) R103.1 R104.1 R105.2 ; also sheet 5,6
Unconnected: IC106.P$2(PD1) IC106.P$12(PE3) IC106.P$13(PE2) IC106.P$14(PE1) IC106.P$15(PE0) IC106.P$18(PK0) IC106.P$19(PK1) IC106.P$20(PK2) IC106.P$21(PK3) IC106.P$22(PC7) IC106.P$23(PC6) IC106.P$24(PC5) IC106.P$25(PC4) IC106.P$31(PH2) IC106.P$32(PH3) IC106.P$42(PF0) IC106.P$43(PF1) IC106.P$46(PF4) IC106.P$53(EN0RXIN) IC106.P$54(EN0RXIP) IC106.P$56(EN0TXON) IC106.P$57(EN0TXOP) IC106.P$60(PK7) IC106.P$65(!HIB) IC106.P$67(XOSC1) IC106.P$71(PM7) IC106.P$72(PM6) IC106.P$73(PM5) IC106.P$74(PM4) IC106.P$75(PM3) IC106.P$76(PM2) IC106.P$102(PQ4) IC106.P$107(PN0) IC106.P$108(PN1) IC106.P$109(PN2) IC106.P$110(PN3) IC106.P$111(PN4) IC106.P$112(PN5) IC106.P$116(PJ0) IC106.P$117(PJ1) IC106.P$118(PP0) IC106.P$119(PP1) IC106.P$121(PB4) IC106.P$123(PE4) IC106.P$124(PE5) IC106.P$125(PD4) IC106.P$126(PD5) IC107.2(NC_2) IC107.4(NC_3) IC107.5(NC) Q101.2(NC) Q101.4(NC2)

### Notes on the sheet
- XDS110 Debug Probe
- R104 and C103 used to meet 
  VBAT rise time requirements
- Texas Instruments

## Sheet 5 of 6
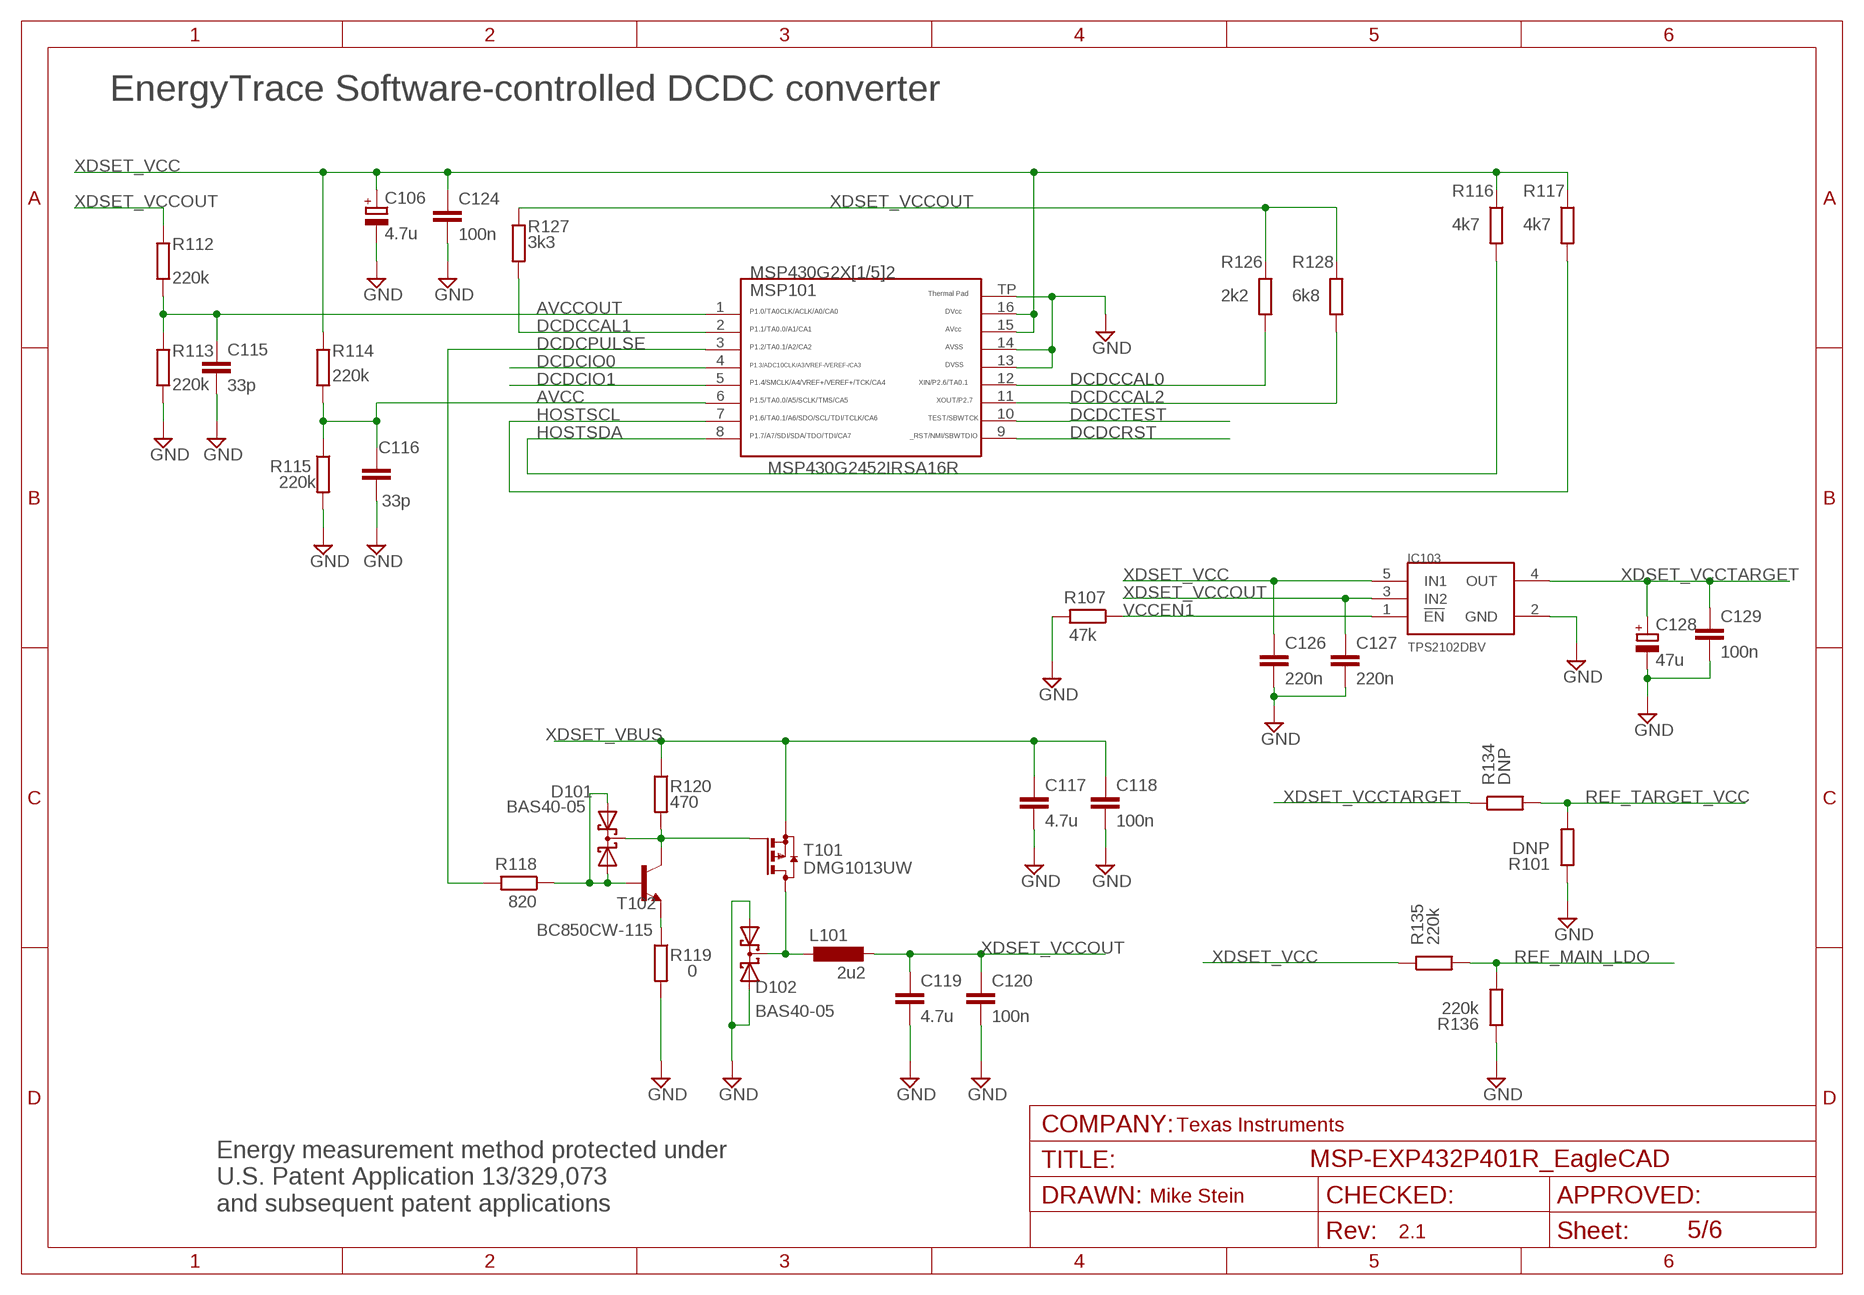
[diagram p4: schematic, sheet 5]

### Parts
C106  4.7u  CPOL-EUA/3216-18R  [A/3216-18R]
C115  33p  C-EUCM0402  [0402]
C116  33p  C-EUCM0402  [0402]
C117  4.7u  C-EUC0603  [C0603]
C118  100n  C-EUCM0402  [0402]
C119  4.7u  C-EUC0603  [C0603]
C120  100n  C-EUCM0402  [0402]
C124  100n  C-EUCM0402  [0402]
C126  220n  C-EUCM0402  [0402]
C127  220n  C-EUCM0402  [0402]
C128  47u  CPOL-EUA/3216-18R  [A/3216-18R]
C129  100n  C-EUCM0402  [0402]
D101  BAS40-05  BAS70-05  [SOT23]
D102  BAS40-05  BAS70-05  [SOT23]
IC103  TPS2102DBV  [SOT23-5]
L101  2u2  L-EUL3216C  [L3216C]
MSP101  MSP430G2452IRSA16R  G2X[1/5]2---RSA16  [RSA16]
R101  DNP  R-EU_RM0402  [0402]
R107  47k  R-EU_RM0402  [0402]
R112  220k  R-EU_RM0402  [0402]
R113  220k  R-EU_RM0402  [0402]
R114  220k  R-EU_RM0402  [0402]
R115  220k  R-EU_RM0402  [0402]
R116  4k7  R-EU_RM0402  [0402]
R117  4k7  R-EU_RM0402  [0402]
R118  820  R-EU_RM0402  [0402]
R119  0  R-EU_RM0402  [0402]
R120  470  R-EU_RM0402  [0402]
R126  2k2  R-EU_RM0402  [0402]
R127  3k3  R-EU_RM0402  [0402]
R128  6k8  R-EU_RM0402  [0402]
R134  DNP  R-EU_RM0402  [0402]
R135  220k  R-EU_RM0402  [0402]
R136  220k  R-EU_RM0402  [0402]
T101  DMG1013UW  BSS84  [SOT23]
T102  BC850CW-115  BC850SMD  [SOT23-BEC]

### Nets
AVCC: C116.2 MSP101.6 R114.2 R115.1
AVCCOUT: C115.2 MSP101.1 R112.2 R113.1
DCDCCAL0: MSP101.12 R126.2
DCDCCAL1: MSP101.2 R127.2
DCDCCAL2: MSP101.11 R128.2
DCDCIO0: MSP101.4 ; also sheet 4
DCDCIO1: MSP101.5 ; also sheet 4
DCDCPULSE: MSP101.3 R118.2 ; also sheet 4
DCDCRST: MSP101.9 ; also sheet 4,6
DCDCTEST: MSP101.10 ; also sheet 4,6
HOSTSCL: MSP101.7 R117.2 ; also sheet 4
HOSTSDA: MSP101.8 R116.2 ; also sheet 4
N$12: R119.1 T102.E
N$13: D101.1(A1) D101.2(A2) R118.1 T102.B
N$15: D102.3(C) L101.1 T101.3(D)
N$16: D101.3(C) R120.2 T101.1(G) T102.C
REF_MAIN_LDO: R135.2 R136.2 ; also sheet 4
REF_TARGET_VCC: R101.2 R134.2 ; also sheet 4
VCCEN1: IC103.1(!EN) R107.1 ; also sheet 4
XDSET_GND: C106.- C115.1 C116.1 C117.2 C118.2 C119.2 C120.2 C124.2 C126.2 C127.2 C128.- C129.2 D102.1(A1) D102.2(A2) IC103.2(GND) MSP101.13 MSP101.14 MSP101.TP R101.1 R107.2 R113.2 R115.2 R119.2 R136.1 ; supply symbol labelled GND ; also sheet 3,4,6
XDSET_VBUS: C117.1 C118.1 R120.1 T101.2(S) ; also sheet 3,4,6
XDSET_VCC: C106.+ C124.1 C126.1 IC103.5(IN1) MSP101.15 MSP101.16 R114.1 R116.1 R117.1 R135.1 ; also sheet 4,6
XDSET_VCCOUT: C119.1 C120.1 C127.1 IC103.3(IN2) L101.2 R112.1 R126.1 R127.1 R128.1
XDSET_VCCTARGET: C128.+ C129.1 IC103.4(OUT) R134.1 ; also sheet 3

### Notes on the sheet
- EnergyTrace Software-controlled DCDC converter
- MSP430G2452IRSA16R
- Texas Instruments
- Energy measurement method protected under 
  U.S. Patent Application 13/329,073 
  and subsequent patent applications

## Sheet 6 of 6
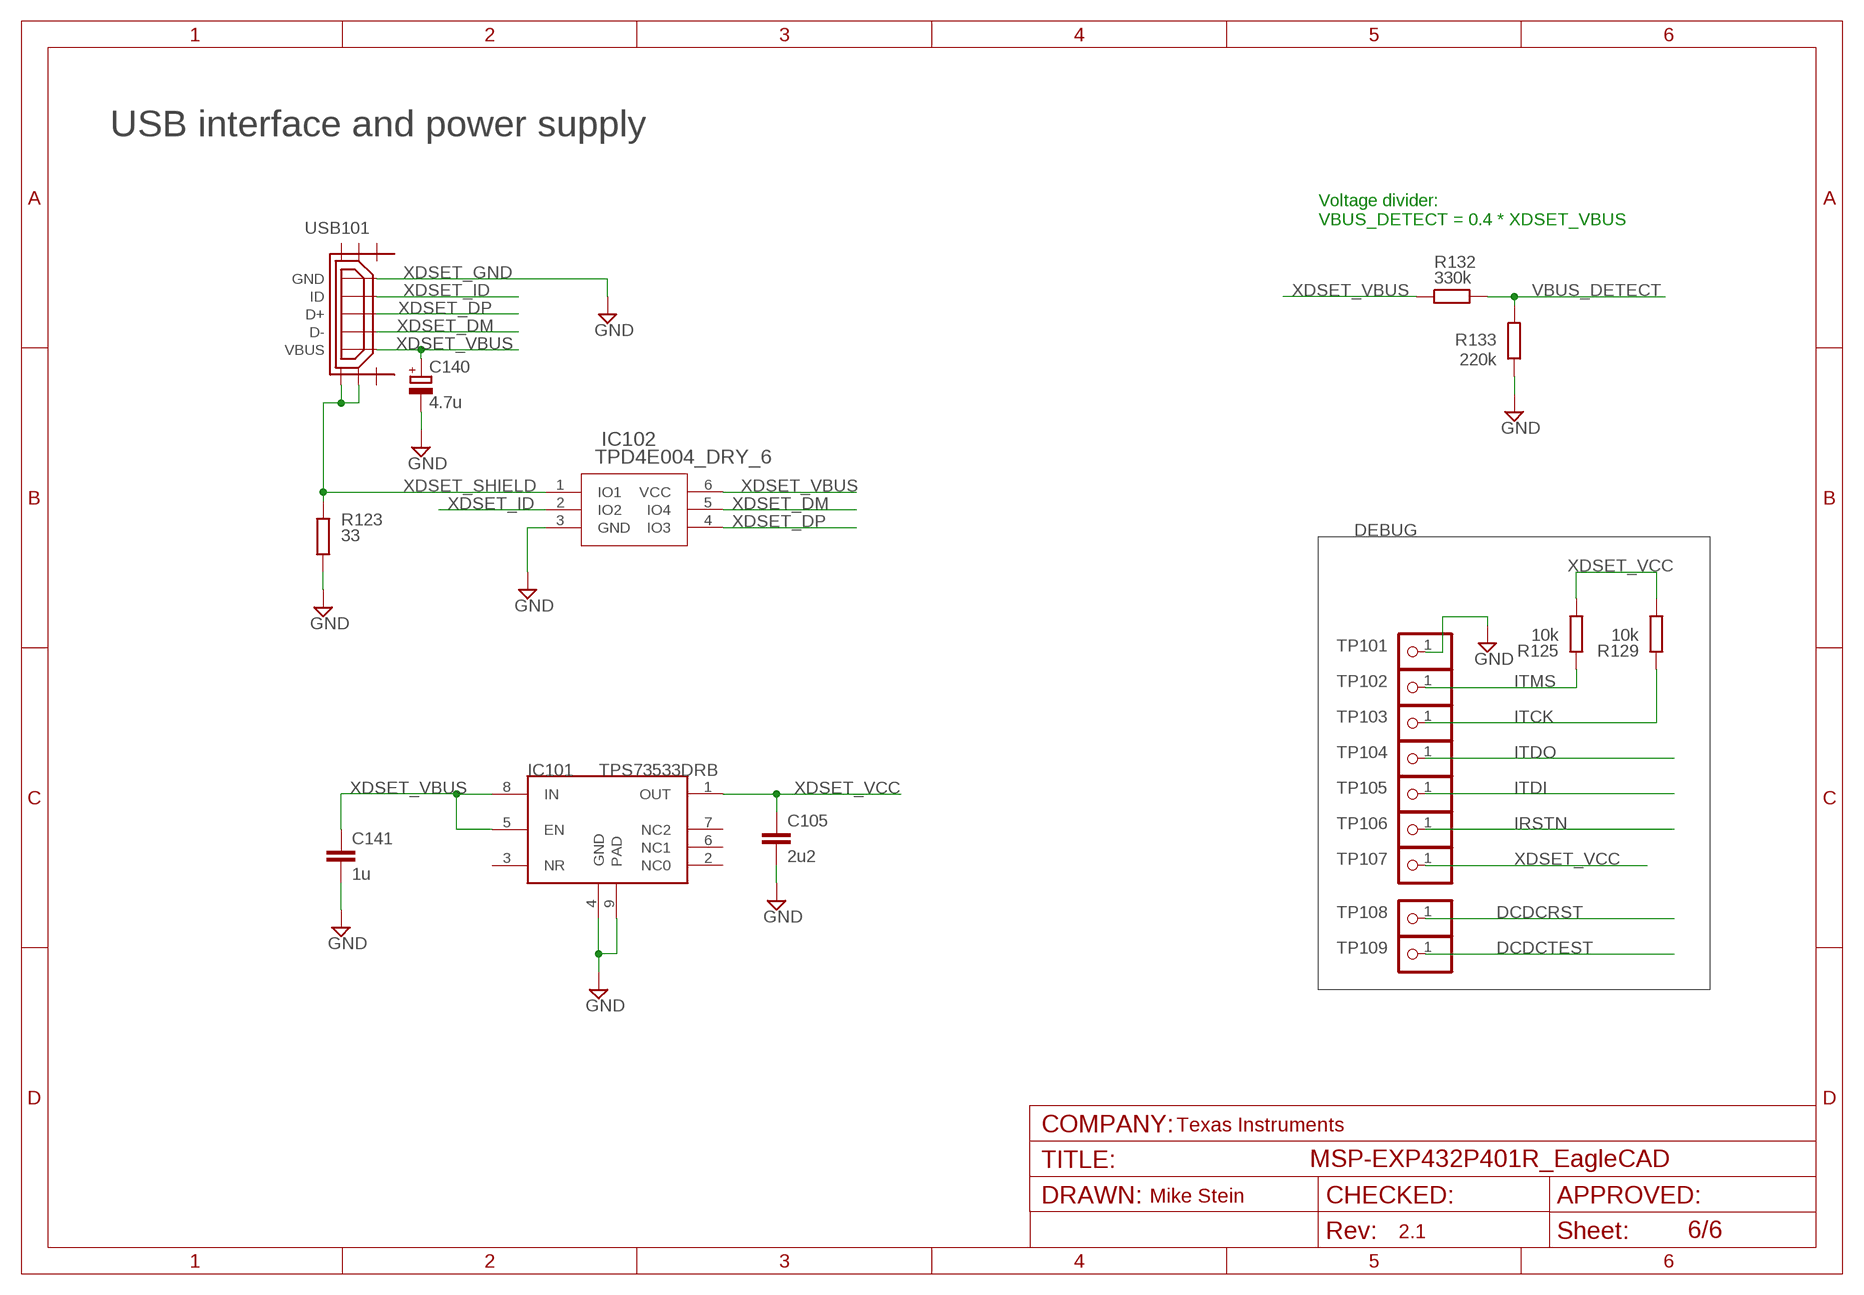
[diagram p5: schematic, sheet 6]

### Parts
C105  2u2  C-EUC0603  [C0603]
C140  4.7u  CPOL-EUA/3216-18R  [A/3216-18R]
C141  1u  C-EUC0603  [C0603]
IC101  TPS73533DRB  TPS73633DRB  [SON8]
IC102  TPD4E004_DRY_6  [DRY6]
R123  33  R-EU_RM0402  [0402]
R125  10k  R-EU_RM0402  [0402]
R129  10k  R-EU_RM0402  [0402]
R132  330k  R-EU_RM0402  [0402]
R133  220k  R-EU_RM0402  [0402]
TP101  TEST_PIN2  PINHD-1X1  [1X01]
TP102  TEST_PIN2  PINHD-1X1  [1X01]
TP103  TEST_PIN2  PINHD-1X1  [1X01]
TP104  TEST_PIN2  PINHD-1X1  [1X01]
TP105  TEST_PIN2  PINHD-1X1  [1X01]
TP106  TEST_PIN2  PINHD-1X1  [1X01]
TP107  TEST_PIN2  PINHD-1X1  [1X01]
TP108  TEST_PIN2  PINHD-1X1  [1X01]
TP109  TEST_PIN2  PINHD-1X1  [1X01]
USB101  USB-MICRO  [MOLEX_105164-0001]

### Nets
DCDCRST: TP108.1 ; also sheet 4,5
DCDCTEST: TP109.1 ; also sheet 4,5
IRSTN: TP106.1 ; also sheet 4
ITCK: R129.1 TP103.1 ; also sheet 4
ITDI: TP105.1 ; also sheet 4
ITDO: TP104.1 ; also sheet 4
ITMS: R125.1 TP102.1 ; also sheet 4
VBUS_DETECT: R132.2 R133.2 ; also sheet 4
XDSET_DM: IC102.5(IO4) USB101.D- ; also sheet 4
XDSET_DP: IC102.4(IO3) USB101.D+ ; also sheet 4
XDSET_GND: C105.2 C140.- C141.2 IC101.4(GND) IC101.9(PAD) IC102.3(GND) R123.2 R133.1 TP101.1 USB101.GND ; supply symbol labelled GND ; also sheet 3,4,5
XDSET_ID: IC102.2(IO2) USB101.ID ; also sheet 4
XDSET_SHIELD: IC102.1(IO1) R123.1 USB101.SHIELD_TH1(SHIELD5) USB101.SHIELD_TH2(SHIELD6)
XDSET_VBUS: C140.+ C141.1 IC101.5(EN) IC101.8(IN) IC102.6(VCC) R132.1 USB101.VBUS ; also sheet 3,4,5
XDSET_VCC: C105.1 IC101.1(OUT) R125.2 R129.2 TP107.1 ; also sheet 4,5
Unconnected: IC101.2(NC0) IC101.3(NR) IC101.6(NC1) IC101.7(NC2) USB101.SHIELD1 USB101.SHIELD2 USB101.SHIELD3 USB101.SHIELD4

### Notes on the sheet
- USB interface and power supply
- Voltage divider:
  VBUS_DETECT = 0.4 * XDSET_VBUS
- DEBUG
- Texas Instruments

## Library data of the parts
C1 C2 C4-C8 C11-C13 C105 C107 C115-C120 C124 C126 C127 C129 C130 C132 C141 = rcl:C-EU: CAPACITOR, European symbol
C3 C106 C128 C140 = rcl:CPOL-EU: POLARIZED CAPACITOR, European symbol
C10 = cap:CSMD0805
C101 C102 = EK-TM4C129EXL:C-US: CAPACITOR, American symbol; GNUM: G10-C0402-C120-AAC
C103 C104 C108 C110-C114 C121 C123 C131 C150 = EK-TM4C129EXL:C-US: CAPACITOR, American symbol; GNUM: G10-C0402-C104-HBA
C133 = EK-TM4C129EXL:C-US: CAPACITOR, American symbol; DIGIKEY_PARTNUM: 311-1451-2-ND; GNUM: G10-C0603-C225-HBB
D101 D102 = diode:BAS70-05: Silicon Schottky Diodes General-purpose diode for high-speed switching
IC101 = MSP430G6_LP:TPS73633DRB
IC102 = MSP-EXP432:TPD4E004_DRY_6; DATASHEETURL: http://www.ti.com/lit/gpn/TPD4E004; DESCRIPTION: 4-Channel ESD Protection Array for High-Speed Data Interfaces; FAMILY_NAME: ESD Solution; GENERIC_PART_NUMBER: TPD4E004; INDUSTRY_STD_PKG_TYPE: SON; MANUFACTURER: Texas Instruments; MANUFACTURER_PART_NUMBER: tpd4e004_dry_6; PACKAGE_DESIGNATOR: DRY; PIN_COUNT: 6; VENDOR: Texas Instruments
IC103 = MSP430G6_LP:TPS2102DBV
IC106 = EK-TM4C129EXL:TM4C129ENCPDT
IC107 = MSP-EXP432:LM4040B25_DCK_5; DATASHEETURL: http://www.ti.com/lit/gpn/LM4040B25; DESCRIPTION: 2.5-V Precision Micropower Shunt Voltage Reference, 0.2% accuracy; FAMILY_NAME: SHUNT VOLTAGE REFERENCE; GENERIC_PART_NUMBER: LM4040B25; INDUSTRY_STD_PKG_TYPE: SC70; MANUFACTURER: Texas Instruments; MANUFACTURER_PART_NUMBER: lm4040b25_dck_5; PACKAGE_DESIGNATOR: DCK; PIN_COUNT: 5; VENDOR: Texas Instruments
J1 = MSP430_Headers:HEADER1X10-J1
J2 = MSP430_Headers:HEADER1X10-J2
J3 = MSP430_Headers:HEADER1X10-J3
J4 = MSP430_Headers:HEADER1X10-J4
J5 = MSP-EXP432:EDGE_CON
J6 = LaunchPad_Template_Library:BP_HEADERS_PWR_3V3; CCO: 258-0001299; DESCRIPTION: CONN HEADER .100 SINGL STR 3POS; MAN: SULLINS
J7 = LaunchPad_Template_Library:BP_HEADERS_PWR_5V
J8 J102 = MSP430_Headers:DEBUG_ARM-10; SAMTEC: FTSH-105-01-F-D-K
J101 = MSP430_Headers:J101_432
JP8-JP11 JP102 = jumper:JP1M
L1 = Murata:LQM2MP_G0
L101 = rcl:L-EU: INDUCTOR, European symbol
LED1 LED101 LED102 = led:LED: LED
LED2 = MSP-EXP432:EVERLIGHT_19-337
MSP1 = MSP-EXP432:MSP432
MSP101 = TI_MSP430_v16:G2X[1/5]2---RSA16: MSP430G2X[1/5]2 MSP430G2x52, MSP430G2x12 QFN (RSA) 16 Pin Package http://focus.ti.com/docs/prod/folders/print/msp430g2452.html
Q1 Q2 = MSP_Crystals:CRYSTAL
Q101 = MSP-EXP432:NX3225GA_OSC
R1-R4 R6 R7 R101 R107 R111-R120 R123-R129 R132-R136 = rcl:R-EU_: RESISTOR, European symbol
R5 = smd:R_0805
R102 R108-R110 = EK-TM4C129EXL:R-US_: RESISTOR, American symbol; GNUM: G11-R0402-1000-AAA
R103 = EK-TM4C129EXL:R-US_: RESISTOR, American symbol; GNUM: G11-R0402-1002-AAA
R104 R105 R131 R137 R138 R140 = EK-TM4C129EXL:R-US_: RESISTOR, American symbol; GNUM: G11-R0402-51R0-AAA
R106 R139 = EK-TM4C129EXL:R-US_: RESISTOR, American symbol; GNUM: G11-R0402-R202-AAA
S1-S3 = MSP430_SwitchesTestpointsJumpers:TS-1188E
T101 = transistor-small-signal:BSS84: P-CHANNEL MOS FET
T102 = transistor-npn:BC850*: NPN Transistor
TP101-TP110 = pinhead:PINHD-1X1: PIN HEADER
U$1-U$3 U$5 = MSP-EXP432:MOUNTHOLE_125MIL
U$7 = Mike:MIKE_TM
U$8 = MSP430_Silkscreen:P401R_REARSILK_REV2_1
U$9 = MSP430_Silkscreen:REAR_TILOGO
U$10 = MSP430_Silkscreen:COMPLIANCE_SUITE
U$11 = MSP430_Silkscreen:COMPLIANCE_FCC_TEXT
U$12 = MSP430_Silkscreen:LOGO-ROCKET
U$13 = MSP-EXP432:P401R_SILKLABEL
USB101 = MSP_Connectors:USB-MICRO

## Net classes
0 default: width 0.254 mm
1 Ground: width 0.203 mm, drill 0.305 mm, clearance 0.152 mm to class 0, clearance 0.152 mm
2 Power: width 0.203 mm, drill 0.305 mm, clearance 0.152 mm to class 0, clearance 0.152 mm to class 1, clearance 0.152 mm

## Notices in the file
MSP-EXP432P401R_EagleCAD.brd:
(C)2003 A. DANNENBERG
